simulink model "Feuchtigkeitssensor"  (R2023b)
settings: Solver=ode1  StartTime=0.0  StopTime=30  FixedStep=0.001  RelTol=1e-3  EnableMultiTasking=on
libraries: arduinolib x2

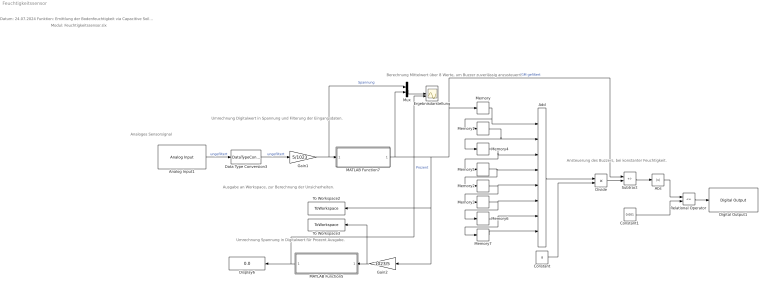
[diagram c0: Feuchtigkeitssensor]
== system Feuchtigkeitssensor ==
  note: Modul: Feuchtigkeitssensor.slx
  note: Datum: 24.07.2024 Funktion: Emittlung der Bodenfeuchtigkeit via Capacitive Soil Moisture Sensor v1.2 Implementierung: Simulink R2023b Toolbox: Simulink Support Package für Arduino Hardware Autor: Ken Hilz Letzte Änderung: 25.07.2024
  note: Analoges Sensorsignal
  note: Ansteuerung des Buzzers, bei konstanter Feuchtigkeit.
  note: Ausgabe an Workspace, zur Berechnung der Unsicherheiten.
  note: Umrechnung Spannung in Digitalwert für Prozent Ausgabe.
  note: Umrechnung Digitalwert in Spannung und Filterung der Eingangsdaten.
  note: Berechnung MIttelwert über 8 Werte, um Buzzer zuverlässig anzusteuern.
  Abs : Abs
  Add : Sum  Inputs=++++++++
  Analog Input1 : arduinolib/Analog Input  pinNumber=0  ReadResultsOnly=off  ConversionTriggerSource=Software  ExternalTriggerType=uint32( 0 )  OutputDataType=uint16  EnableConversionCompleteNotify=off  EnableOuputStatus=off  SampleTime=-1  blockPlatform=arduino
  Constant : Constant  Value=8
  Constant1 : Constant  Value=0.001
  Data Type Conversion3 : DataTypeConversion  OutDataTypeStr=double
  Digital Output1 : arduinolib/Digital Output  pinNumber=10  Direction=output  blockPlatform=arduino
  Display6 : Display
  Divide : Product  Inputs=*/
  Ergebnisdarstellung : Scope  NumInputPorts=2
  Gain1 : Gain  Gain=5/1023
  Gain2 : Gain  Gain=1023/5
  MATLAB Function5 : MATLAB Function  TreatAsAtomicUnit=on
  MATLAB Function7 : MATLAB Function  TreatAsAtomicUnit=on
  Memory{,1..7} (8 alike) : Memory
  Mux : Mux  Inputs=2
  Relational Operator : RelationalOperator  Operator=<=  OutDataTypeStr=boolean  RndMeth=Simplest
  Subtract : Sum  Inputs=+-
  To Workspace2 : ToWorkspace  VariableName=Voltage  SampleTime=-1
  To Workspace3 : ToWorkspace  VariableName=Digitalwert  SampleTime=-1
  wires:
  Analog Input1/1 -> Data Type Conversion3/1  "ungefiltert"
  MATLAB Function5/1(Prozent) -> Ergebnisdarstellung/2, Display6/1  "Prozent"
  Data Type Conversion3/1 -> Gain1/1  "ungefiltert"
  MATLAB Function7/1(RGM) -> Mux/2, Gain2/1, To Workspace2/1, Memory/1, Subtract/1  "RGM gefiltert"
  Gain1/1 -> Mux/1, MATLAB Function7/1(x)  "Spannung"
  Gain2/1 -> To Workspace3/1, MATLAB Function5/1(Digitalwert)
  Memory/1 -> Memory1/1, Add/1
  Memory1/1 -> Memory4/1, Add/2
  Memory4/1 -> Memory5/1, Add/3
  Memory5/1 -> Memory2/1, Add/4
  Memory2/1 -> Memory3/1, Add/5
  Memory3/1 -> Memory6/1, Add/6
  Memory6/1 -> Memory7/1, Add/7
  Memory7/1 -> Add/8
  Constant/1 -> Divide/2
  Add/1 -> Divide/1
  Divide/1 -> Subtract/2
  Subtract/1 -> Abs/1
  Relational Operator/1 -> Digital Output1/1
  Constant1/1 -> Relational Operator/2
  Abs/1 -> Relational Operator/1
  Mux/1 -> Ergebnisdarstellung/1

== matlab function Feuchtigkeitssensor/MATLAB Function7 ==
function RGM = RekGleitenderMittelwert(x)

persistent n aSchieberegister
persistent bErsterDurchlauf

if isempty (bErsterDurchlauf)
    n=160;
    aSchieberegister = x* ones (n,1);
    bErsterDurchlauf = 1;
end

for m=1:n-1
    aSchieberegister (m) = aSchieberegister (m+1);
end

aSchieberegister (n) = x;
RGM = x;

RGM = sum(aSchieberegister)/n;
end

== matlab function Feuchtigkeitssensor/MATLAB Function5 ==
function Prozent = DigitalwertinProzent(Digitalwert)
    % Bestimmung des aktuellen Digitalwertes
    max_Digitalwert = 789; % maximaler Digitalwert, der vom Sensor ausgegeben wird
    min_Digitalwert = 388; % minimaler Digitalwert, der vom Sensor ausgegeben wird
    Grundwert = max_Digitalwert-min_Digitalwert; % Bestimmung des Werte Bereichs, dass 0-100% bestimmt
    akt_Digitalwert = Digitalwert-min_Digitalwert;  % ADC resolution (for Arduino Uno, assuming 10-bit)

    % Umrechnung des Digitalwertes in Prozent
    Prozent = (1-(akt_Digitalwert/Grundwert))*100;
end
